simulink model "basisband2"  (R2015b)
settings: Solver=VariableStepAuto  StartTime=0.0  StopTime=10.0  RelTol=1e-3
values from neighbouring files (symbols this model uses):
  ampl1 = 1    [basisband_2.m]    (also in ad_test_2.m = 0.0001; ad_test_3.m = 0.0001; DA_wandler_spektr_1.m; DA_wandler_spektr_2.m)
  ampl2 = 0.5    [basisband_2.m]    (also in ad_test_2.m = 1e-05; ad_test_3.m = 1e-05; DA_wandler_spektr_1.m = 1; DA_wandler_spektr_2.m = 1)
  delay = 2*nord1/2 + (nord2/2)*M1-1    (= 1535)    [basisband_2.m]    (also in ifir_dezim_1.m = fix((length(himage)-1)/2 + 5*(length(h)-1)/2); ifir_high_2.m = length(d)-1; ifir_interp_1.m = fix((length(h)-1)/2 + (length(himage)-1)/(2*L)))
  delta_f1 = 200    [basisband_1.m]    (also in basisband_2.m)
  delta_f2 = 250    [basisband_1.m]    (also in basisband_2.m = 300)
  f0 = 5000    [basisband_1.m]    (also in basisband_2.m = 40000; mehrdeutigkeit_1.m = 200; spektr_pulse_1.m = 1010)
  hdez1 = fir1(nord1, 1/M1)    [basisband_2.m]
  hdez2 = fir1(nord2, fp2)    [basisband_2.m]
  hnoise = fir1(nord0, fnoise)    [basisband_2.m]
  M1 = 20    [basisband_2.m]
  noise = 0.5    [basisband_2.m]    (also in farrow_2.m = randn(1,nt); farrow_3.m = randn(1,nt);     rng(s); farrow_4.m = randn(1,nt);     rng(s); leakage_4.m = 2)
  Ts = 1/fs    (= 5e-05)    [basisband_1.m]    (also in basisband_2.m = 5e-06; dezimier_1.m = 0.0005; dezimier_11.m = 0.0005; dezimier_2.m = 0.0005)
libraries: simulink x1, dspsrcs4 x1, dspsigops x1, dspstat3 x1

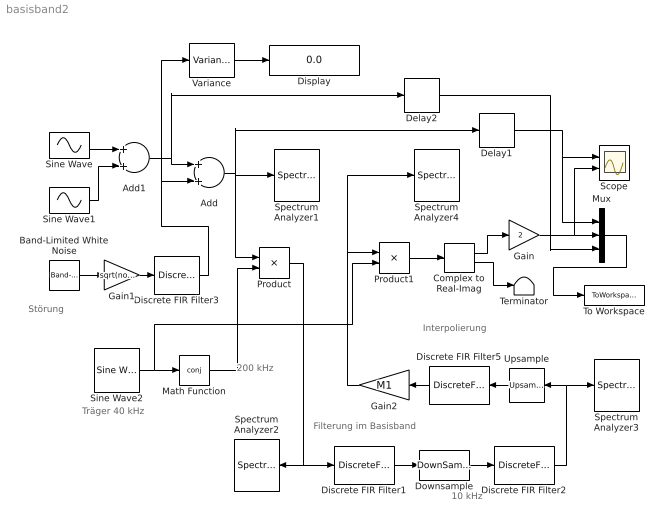
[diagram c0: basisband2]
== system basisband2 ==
  note: Interpolierung
  note: Störung
  note: Träger 40 kHz
  note: 10 kHz
  note: 200 kHz
  note: Filterung im Basisband
  Add : Sum
  Add1 : Sum
  Band-Limited White Noise : simulink/Sources/Band-Limited White Noise  Cov=Ts  Ts=Ts  seed=[23341]
  Complex to Real-Imag : ComplexToRealImag
  Delay1 : Delay  DelayLength=delay
  Delay2 : Delay  DelayLength=delay
  Discrete FIR Filter1 : DiscreteFir  Coefficients=hdez1  SampleTime=Ts
  Discrete FIR Filter2 : DiscreteFir  Coefficients=hdez2  SampleTime=Ts*M1
  Discrete FIR Filter3 : DiscreteFir  Coefficients=hnoise  SampleTime=Ts
  Discrete FIR Filter5 : DiscreteFir  Coefficients=hdez1  SampleTime=Ts
  Display : Display
  Downsample : DownSample  N=M1  RateOptions=Allow multirate processing
  Gain : Gain  Gain=2
  Gain1 : Gain  Gain=sqrt(noise)
  Gain2 : Gain  Gain=M1
  Math Function : Math  Operator=conj
  Mux : Mux  Inputs=3
  Product : Product
  Product1 : Product
  Scope : Scope  NumInputPorts=2
  Sine Wave : Sin  Amplitude=ampl1  Frequency=2*pi*(f0+delta_f1)  SampleTime=Ts
  Sine Wave1 : Sin  Amplitude=ampl2  Frequency=2*pi*(f0-delta_f2)  SampleTime=Ts
  Sine Wave2 : dspsrcs4/Sine Wave  Amplitude=1  Frequency=f0  Phase=0  SampleMode=Discrete  OutComplex=Complex  CompMethod=Trigonometric fcn  TableSize=Speed  SampleTime=Ts  SamplesPerFrame=1  ResetState=Restart at time zero  OutputFrames=off  dataType=double  wordLen=16  udDataType=sfix(16)  fracBitsMode=Best precision  numFracBits=15  OutDataTypeStr=double  LastOutDataTypeStr=double
  Spectrum Analyzer{1..4} (4 alike) : SpectrumAnalyzer
  Terminator : Terminator
  To Workspace : ToWorkspace  VariableName=y  SaveFormat=Timeseries  SampleTime=-1
  Upsample : dspsigops/Upsample  N=M1  phase=0  RateOptions=Allow multirate processing  ic=0  mode=Unused parameter value
  Variance : dspstat3/Variance  run=on  reset_popup=None  InputProcessing=Columns as channels (frame based)  directionMode=Each column  dimension=1  roiEnable=off  roiType=Rectangles  roiPortion=Entire ROI  roiOutput=Individual statistics for each ROI  roiFlag=off  roundingMode=Floor  overflowMode=off
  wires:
  Math Function/1 -> Product/2
  Product/1 -> Spectrum Analyzer2/1, Discrete FIR Filter1/1
  Sine Wave2/1 -> Product1/2, Math Function/1
  Product1/1 -> Complex to Real-Imag/1
  Gain/1 -> Scope/2, Mux/2
  Add/1 -> Spectrum Analyzer1/1, Product/1, Delay1/1
  Band-Limited White Noise/1 -> Gain1/1
  Gain1/1 -> Discrete FIR Filter3/1
  Complex to Real-Imag/1 -> Gain/1
  Complex to Real-Imag/2 -> Terminator/1
  Delay1/1 -> Scope/1, Mux/1
  Discrete FIR Filter1/1 -> Downsample/1
  Downsample/1 -> Discrete FIR Filter2/1
  Mux/1 -> To Workspace/1
  Discrete FIR Filter3/1 -> Add/2, Variance/1
  Sine Wave1/1 -> Add1/2
  Sine Wave/1 -> Add1/1
  Add1/1 -> Delay2/1, Add/1
  Delay2/1 -> Mux/3
  Gain2/1 -> Spectrum Analyzer4/1, Product1/1
  Discrete FIR Filter2/1 -> Upsample/1, Spectrum Analyzer3/1
  Upsample/1 -> Discrete FIR Filter5/1
  Variance/1 -> Display/1
  Discrete FIR Filter5/1 -> Gain2/1
